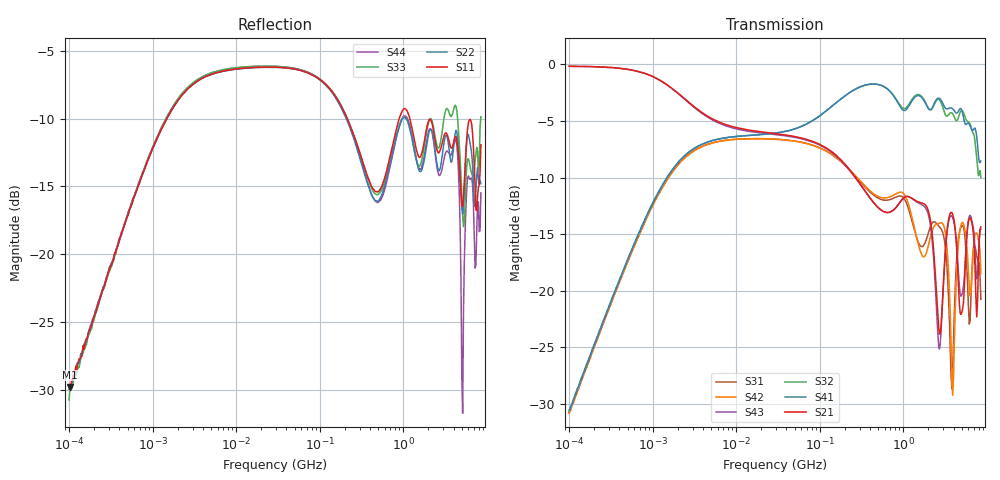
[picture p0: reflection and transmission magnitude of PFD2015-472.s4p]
# MHz S MA R 50
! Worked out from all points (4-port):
!   498 points, 100 kHz to 8.5 GHz, reference 50 ohm
!   strongest paths, dB at 100 kHz, 1.698 MHz, 29.49 MHz, 500.7 MHz, 8.5 GHz:
!     S21: -0.2, -2.1, -6.1, -12.6, -14.3
!     S41: -30.5, -9.4, -6.1, -1.8, -8.5
!     S32: -30.6, -9.4, -6.1, -1.8, -10.0
!     S43: -0.2, -2.1, -6.2, -12.6, -14.6
!     S42: -30.8, -9.6, -6.6, -11.7, -18.5
!     S31: -30.7, -9.6, -6.6, -11.8, -20.8
!   lowest |S11| = -29.8 dB at 102.3 kHz (marker M1), VSWR 1.07, Z = 51.4 + j2.97 ohm
!   |S11| at or under -10 dB: start of sweep to 1.482 MHz; 213.2 MHz to 895.4 MHz (682.2 MHz wide, 123 % of centre); 1.198 GHz to end of sweep
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0.1  0.03297 63.9  0.9814 -1.7  0.02907 -94.4  0.0298 85.7
     0.9814 -1.7  0.03171 66.6  0.02949 85.0  0.02879 -94.9
     0.02907 -94.4  0.02949 85.0  0.02898 63.6  0.9823 -1.7
     0.0298 85.7  0.02879 -94.9  0.9823 -1.7  0.03237 67.4
0.1023101  0.03239 63.2  0.9815 -1.8  0.02939 -94.5  0.03006 85.6
           0.9815 -1.8  0.03246 67.4  0.03022 85.5  0.02933 -94.7
           0.02939 -94.5  0.03022 85.5  0.03195 64.4  0.9811 -1.8
           0.03006 85.6  0.02933 -94.7  0.9811 -1.8  0.03126 66.8
252.3442  0.2778 -65.1  0.327 -98.2  0.3282 81.5  0.7685 -21.9
          0.327 -98.2  0.2704 -67.0  0.7688 -22.1  0.33 79.3
          0.3282 81.5  0.7688 -22.1  0.2774 -64.4  0.3246 -98.2
          0.7685 -21.9  0.33 79.3  0.3246 -98.2  0.2747 -67.6
1431.488  0.244 151.3  0.2492 -89.2  0.1739 95.8  0.7246 174.2
          0.2492 -89.2  0.2231 151.0  0.7326 171.8  0.1748 103.2
          0.1739 95.8  0.7326 171.8  0.2225 149.8  0.2476 -89.8
          0.7246 174.2  0.1748 103.2  0.2476 -89.8  0.2263 150.9
2652.059  0.2359 20.5  0.06921 -73.8  0.1937 95.2  0.7094 13.8
          0.06921 -73.8  0.2034 14.2  0.7006 8.6  0.1983 95.5
          0.1937 95.2  0.7006 8.6  0.2464 2.0  0.05714 -86.3
          0.7094 13.8  0.1983 95.5  0.05714 -86.3  0.1966 15.7
4092.906  0.2653 -148.1  0.2007 -115.8  0.08092 -14.7  0.6229 -176.2
          0.2007 -115.8  0.2657 -142.7  0.5841 179.3  0.06046 -14.6
          0.08092 -14.7  0.5841 179.3  0.3497 -160.3  0.1965 -115.4
          0.6229 -176.2  0.06046 -14.6  0.1965 -115.4  0.2599 -150.6
8500  0.2531 -24.2  0.1917 47.6  0.0917 13.8  0.3753 -32.1
      0.1917 47.6  0.1819 -40.2  0.3164 -41.4  0.1194 -13.4
      0.0917 13.8  0.3164 -41.4  0.3209 -55.9  0.1871 30.3
      0.3753 -32.1  0.1194 -13.4  0.1871 30.3  0.1683 -19.4
